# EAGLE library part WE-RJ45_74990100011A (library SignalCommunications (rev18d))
Order Code 74990100011A Design THT xBase-T 10/100 Base-T Ports 1x1 Application Standard Tab Position UP LED (Left-Right) NONE EMI Fingers No Details see: http://katalog.we-online.de/en/pbs/WE-LAN_RJ45/74990100011A? Updated by Yingchun Shan 2016-08-23 2014 (C) Würth Elektronik
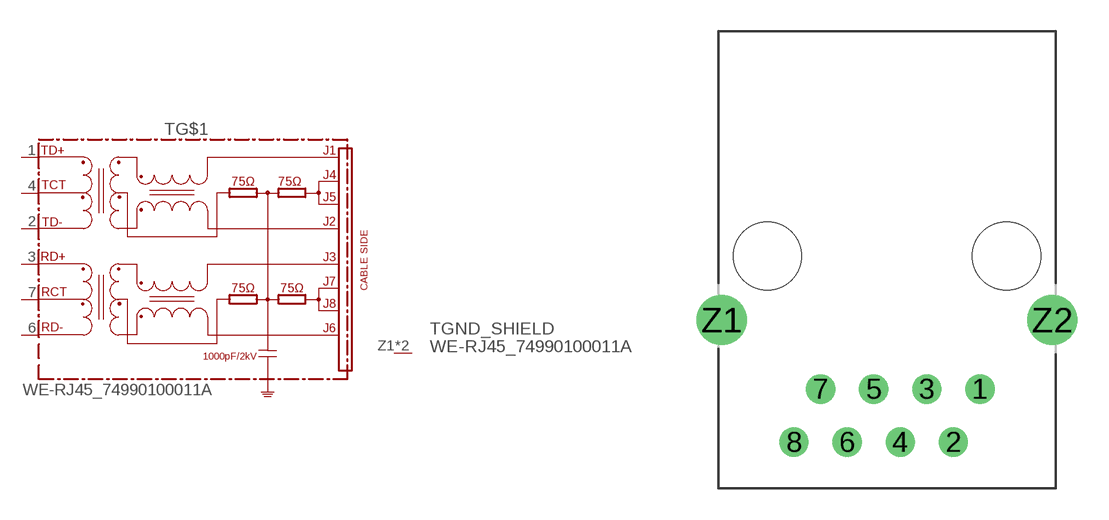
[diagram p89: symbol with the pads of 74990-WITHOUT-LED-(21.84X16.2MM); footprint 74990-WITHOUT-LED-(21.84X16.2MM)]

Designator prefix T; gates GND_SHIELD=GNDPIN G$1=74990100011A

## WE-RJ45_74990100011A (COMPANY-URL: http://www.we-online.de; CREATED-BY: Christin Zierenner; CREATED-DATE: AUG 2012; DATASHEET-URL: http://katalog.we-online.de/kataloge/eisos/media/pdf/74990100011A.pdf; MANUFACTURER: Würth Elektronik eiSos GmbH)  [74990-WITHOUT-LED-(21.84X16.2MM)]
1  G$1:TD+
2  G$1:TD-
3  G$1:RD+
4  G$1:TCT
6  G$1:RD-
7  G$1:RCT
Z1  GND_SHIELD:GND  pwr
Z2  GND_SHIELD:GND  pwr

## Footprint 74990-WITHOUT-LED-(21.84X16.2MM) (pad centres in mm)
MAX HEIGHT=13.74mm PORTS----1X1 LED ----NO
drill 0.89: 1 4.445,-6.35; 2 3.175,-8.89; 3 1.905,-6.35; 4 0.635,-8.89; 5 -0.635,-6.35; 6 -1.905,-8.89; 7 -3.175,-6.35; 8 -4.445,-8.89
drill 1.6: Z1 -7.9,-3.05; Z2 7.9,-3.05
hole 3.25 at 5.715,0
hole 3.25 at -5.715,0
